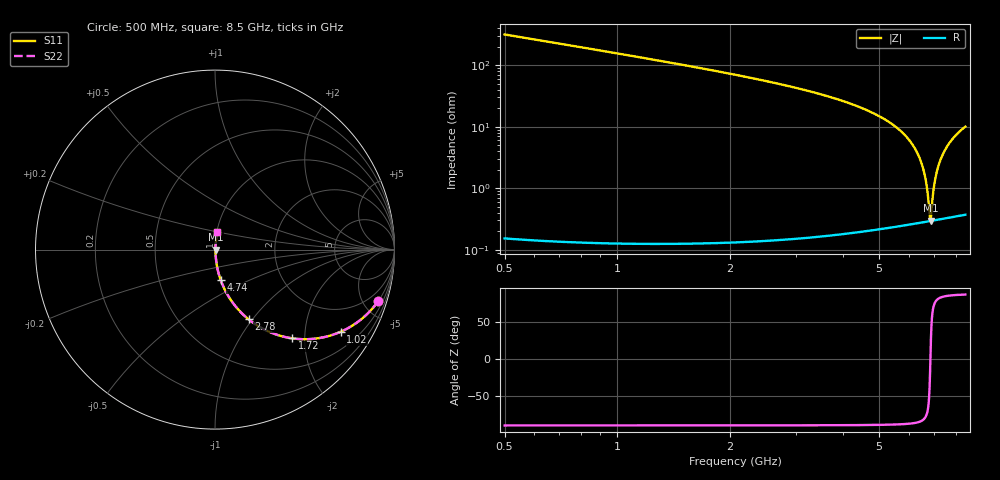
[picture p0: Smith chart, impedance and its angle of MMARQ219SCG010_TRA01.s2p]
! MMARQ219SCG010_TRA01  S-PARAMETER MODEL  ( General Type )
! Model Generated by TAIYO YUDEN Corporation (http://www.ty-top.com)
! Version 1.0
! TAIYO YUDEN Control No. 180601
! Copyright(c) 2018 TAIYO YUDEN CO.,LTD. All Rights Reserved.
! Product Description (link to TY-COMPAS)
! https://ds.yuden.co.jp/TYCOMPAS/or/detail?pn=MMARQ219SCG010BTRA01&u=M
! Products Name : Multilayer Ceramic Capacitors
! Characteristics :
!  Capacitance : 1 pF , Rated Voltage : 250V , TCC : CG / C0G
!  Case Size : 2.0 x 1.25 / 0.079 x 0.049 [mm/inch] , Thickness : 0.85 / 0.033 [mm/inch]
!  (Conditions: Temperature = 25 degC , DC Bias Current/Voltage = 0A / 0V)
! External Node Assignments :
!  1  o---| |---o  2
! GND o---------o GND
! Frequency Range : 500MHz  -  8500MHz  [ 401 STEP ]
# MHz S RI R 50
! Freq[MHz].  S11 Real  S11 Imag  S21 Real  S21 Imag  S12 Real  S12 Imag  S22 Real  S22 Imag
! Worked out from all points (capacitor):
!   401 points, 500 MHz to 8.5 GHz, reference 50 ohm
!   read as one part in series: C = 998 fF near 540 MHz
!   lowest |Z| = 296 mohm at 6.86 GHz (marker M1)
!   series resonance near 6.854 GHz, so ESL is about 540 pH
!   S11 on the Smith chart (normalised r, x): 500 MHz: 1.00, -6.34; 1.02 GHz: 1.00, -3.06; 1.72 GHz: 1.00, -1.74; 2.78 GHz: 1.00, -0.96; 4.74 GHz: 1.00, -0.35; 8.5 GHz: 1.01, +0.20
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500  0.9095 -0.2867  0.0905 0.2867  0.0905 0.2867  0.9095 -0.2867
1020  0.7001 -0.4578  0.2999 0.4578  0.2999 0.4578  0.7001 -0.4578
1720  0.43 -0.4943  0.57 0.4943  0.57 0.4943  0.43 -0.4943
1840  0.3927 -0.4876  0.6073 0.4876  0.6073 0.4876  0.3927 -0.4876
2780  0.1873 -0.3886  0.8127 0.3886  0.8127 0.3886  0.1873 -0.3886
3180  0.1349 -0.3396  0.8651 0.3396  0.8651 0.3396  0.1349 -0.3396
4500  0.0407 -0.1928  0.9593 0.1928  0.9593 0.1928  0.0407 -0.1928
4740  0.0317 -0.1694  0.9683 0.1694  0.9683 0.1694  0.0317 -0.1694
5840  0.00798 -0.0739  0.992 0.0739  0.992 0.0739  0.00798 -0.0739
6240  0.00453 -0.0433  0.9955 0.0433  0.9955 0.0433  0.00453 -0.0433
6520  0.0033 -0.0231  0.9967 0.0231  0.9967 0.0231  0.0033 -0.0231
6680  0.00298 -0.0119  0.997 0.0119  0.997 0.0119  0.00298 -0.0119
6740  0.00293 -0.00776  0.9971 0.00776  0.9971 0.00776  0.00293 -0.00776
6820  0.00291 -0.00231  0.9971 0.00231  0.9971 0.00231  0.00291 -0.00231
6860  0.00292 0.000384  0.9971 -0.000384  0.9971 -0.000384  0.00292 0.000384
6880  0.00293 0.00173  0.9971 -0.00173  0.9971 -0.00173  0.00293 0.00173
6960  0.00302 0.00706  0.997 -0.00706  0.997 -0.00706  0.00302 0.00706
7020  0.00312 0.011  0.9969 -0.011  0.9969 -0.011  0.00312 0.011
7180  0.00353 0.0214  0.9965 -0.0214  0.9965 -0.0214  0.00353 0.0214
7400  0.00442 0.0353  0.9956 -0.0353  0.9956 -0.0353  0.00442 0.0353
7680  0.00606 0.0524  0.9939 -0.0524  0.9939 -0.0524  0.00606 0.0524
8500  0.0136 0.0988  0.9864 -0.0988  0.9864 -0.0988  0.0136 0.0988
